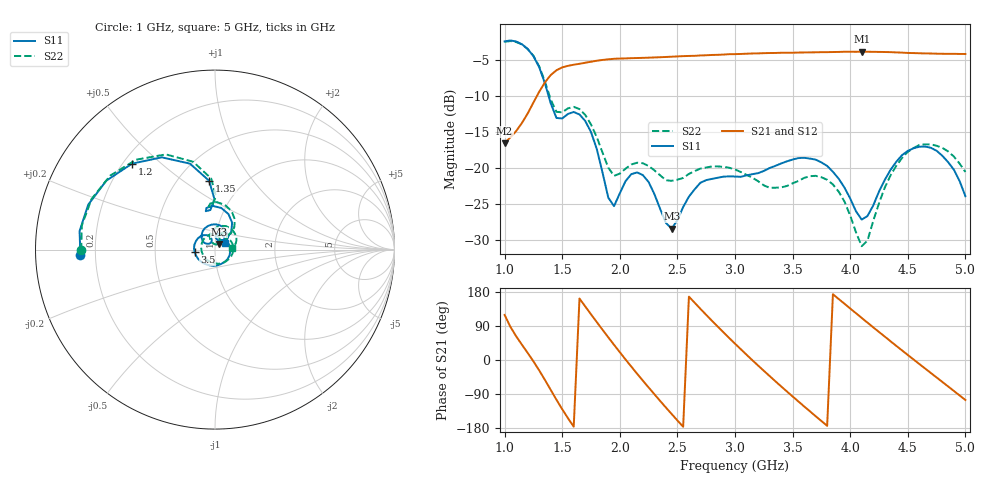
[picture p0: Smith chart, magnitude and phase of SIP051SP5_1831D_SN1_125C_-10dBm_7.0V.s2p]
# GHz  S  dB  R  50
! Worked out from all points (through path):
!   81 points, 1 GHz to 5 GHz, reference 50 ohm
!   highest |S21| = -3.92 dB at 4.1 GHz (marker M1); lowest = -16.6 dB at 1 GHz (marker M2)
!   lowest |S11| = -28.4 dB at 2.45 GHz (marker M3), VSWR 1.08, Z = 52.2 + j3.23 ohm
!   |S11| at or under -10 dB: 1.381 GHz to end of sweep
!   |S22| runs from -30.8 to -2.5 dB; largest |S21 - S12| = 0.0023
!   S11 on the Smith chart (normalised r, x): 1 GHz: 0.14, -0.02; 1.2 GHz: 0.24, +0.40; 1.35 GHz: 0.70, +0.63; 3.5 GHz: 0.80, -0.02; 5 GHz: 1.11, +0.08
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1  -2.49 -177.7  -16.57 119.1  -16.58 119.0  -2.55 -179.8
1.2  -3.54 134.0  -12.47 18.8  -12.46 18.8  -3.53 131.2
1.35  -8.29 94.9  -8.16 -52.6  -8.14 -52.6  -8.04 93.1
1.5  -13.15 103.5  -6.08 -129.9  -6.08 -129.8  -12.30 98.4
1.7  -13.49 69.2  -5.45 141.3  -5.44 141.3  -12.66 66.3
1.85  -20.62 43.1  -5.05 79.8  -5.05 79.8  -17.85 45.7
1.95  -25.26 74.1  -4.90 40.0  -4.91 40.0  -21.07 59.4
2.05  -21.80 86.9  -4.85 1.3  -4.86 1.4  -20.08 68.5
2.2  -20.97 57.8  -4.77 -54.4  -4.76 -54.3  -19.33 54.3
2.35  -25.63 37.6  -4.68 -107.9  -4.67 -107.9  -21.00 44.0
2.45  -28.37 54.2  -4.61 -142.5  -4.61 -142.5  -21.76 44.3
2.6  -23.95 58.0  -4.51 167.2  -4.50 167.3  -20.81 41.4
2.75  -21.66 22.7  -4.41 119.1  -4.40 119.2  -19.92 24.9
3  -21.17 -51.4  -4.25 43.1  -4.24 43.1  -20.19 -21.6
3.2  -20.71 -106.8  -4.15 -14.5  -4.14 -14.4  -21.81 -76.3
3.5  -18.82 -173.0  -4.06 -96.2  -4.06 -96.2  -22.11 171.0
3.7  -18.83 146.7  -4.00 -148.2  -3.99 -148.3  -21.07 111.4
3.9  -21.46 113.9  -3.95 161.0  -3.94 161.0  -23.25 68.3
4.1  -27.12 121.1  -3.92 110.9  -3.90 111.0  -30.79 75.7
4.35  -20.25 139.5  -3.98 49.5  -4.00 49.5  -21.01 107.3
4.65  -17.03 88.1  -4.16 -22.4  -4.17 -22.5  -16.73 56.2
5  -23.88 32.2  -4.24 -105.5  -4.24 -105.5  -20.54 4.8
